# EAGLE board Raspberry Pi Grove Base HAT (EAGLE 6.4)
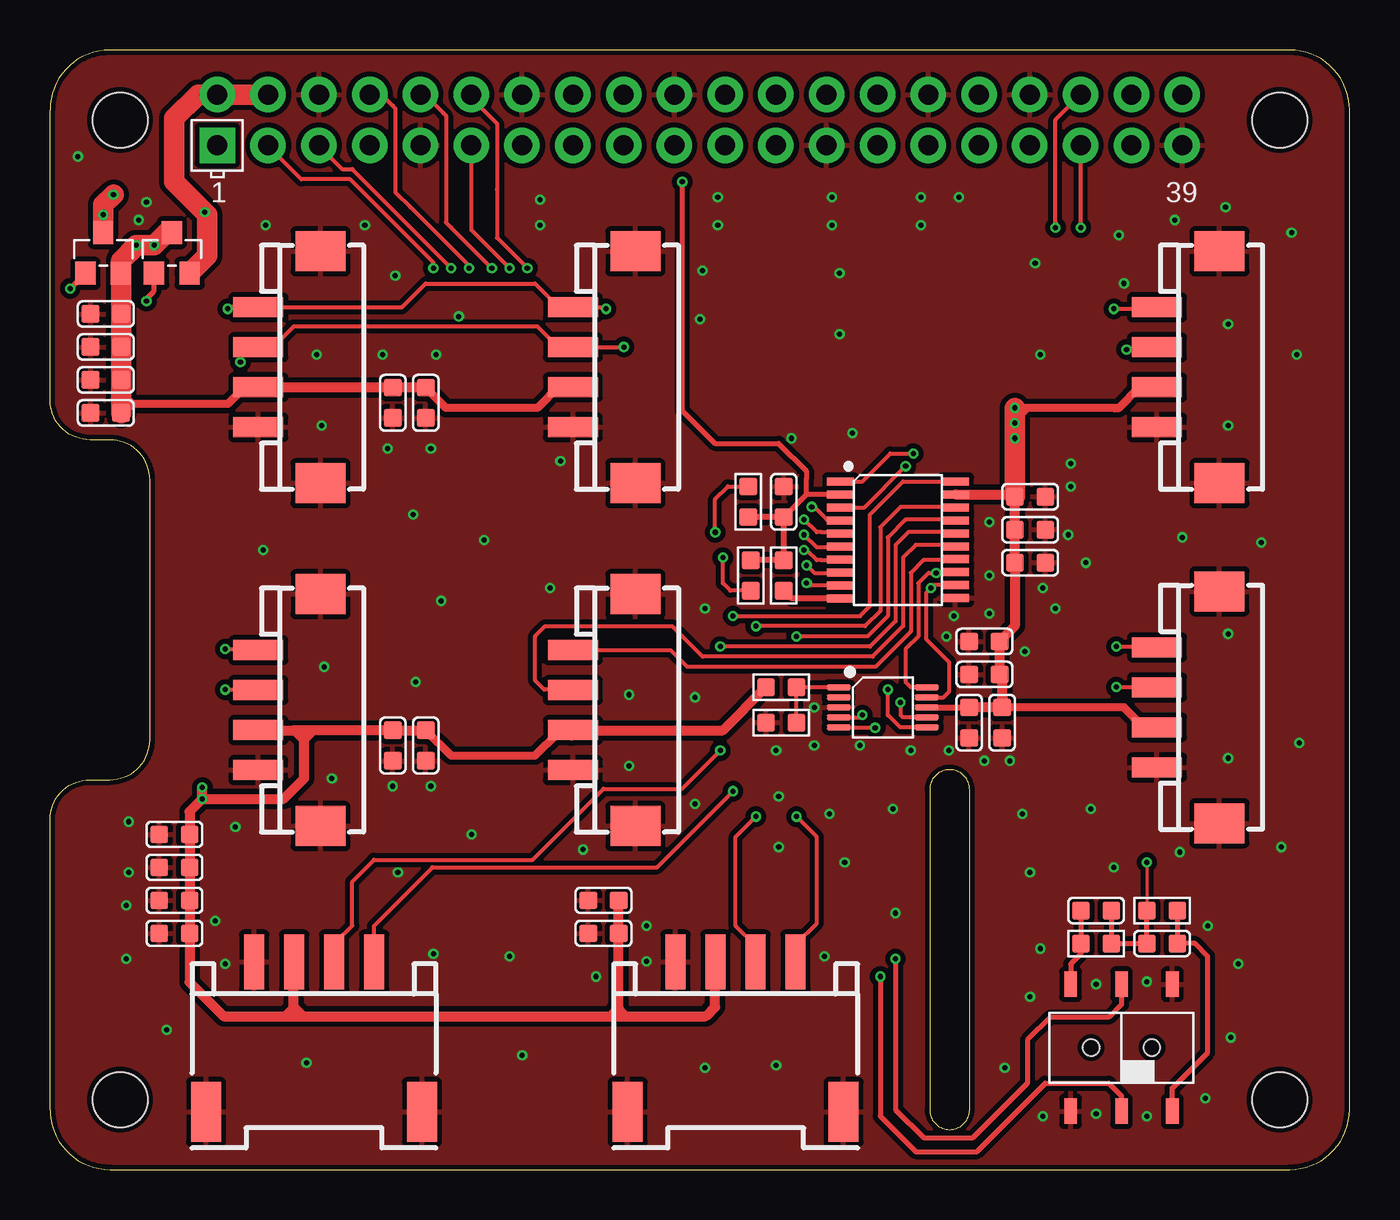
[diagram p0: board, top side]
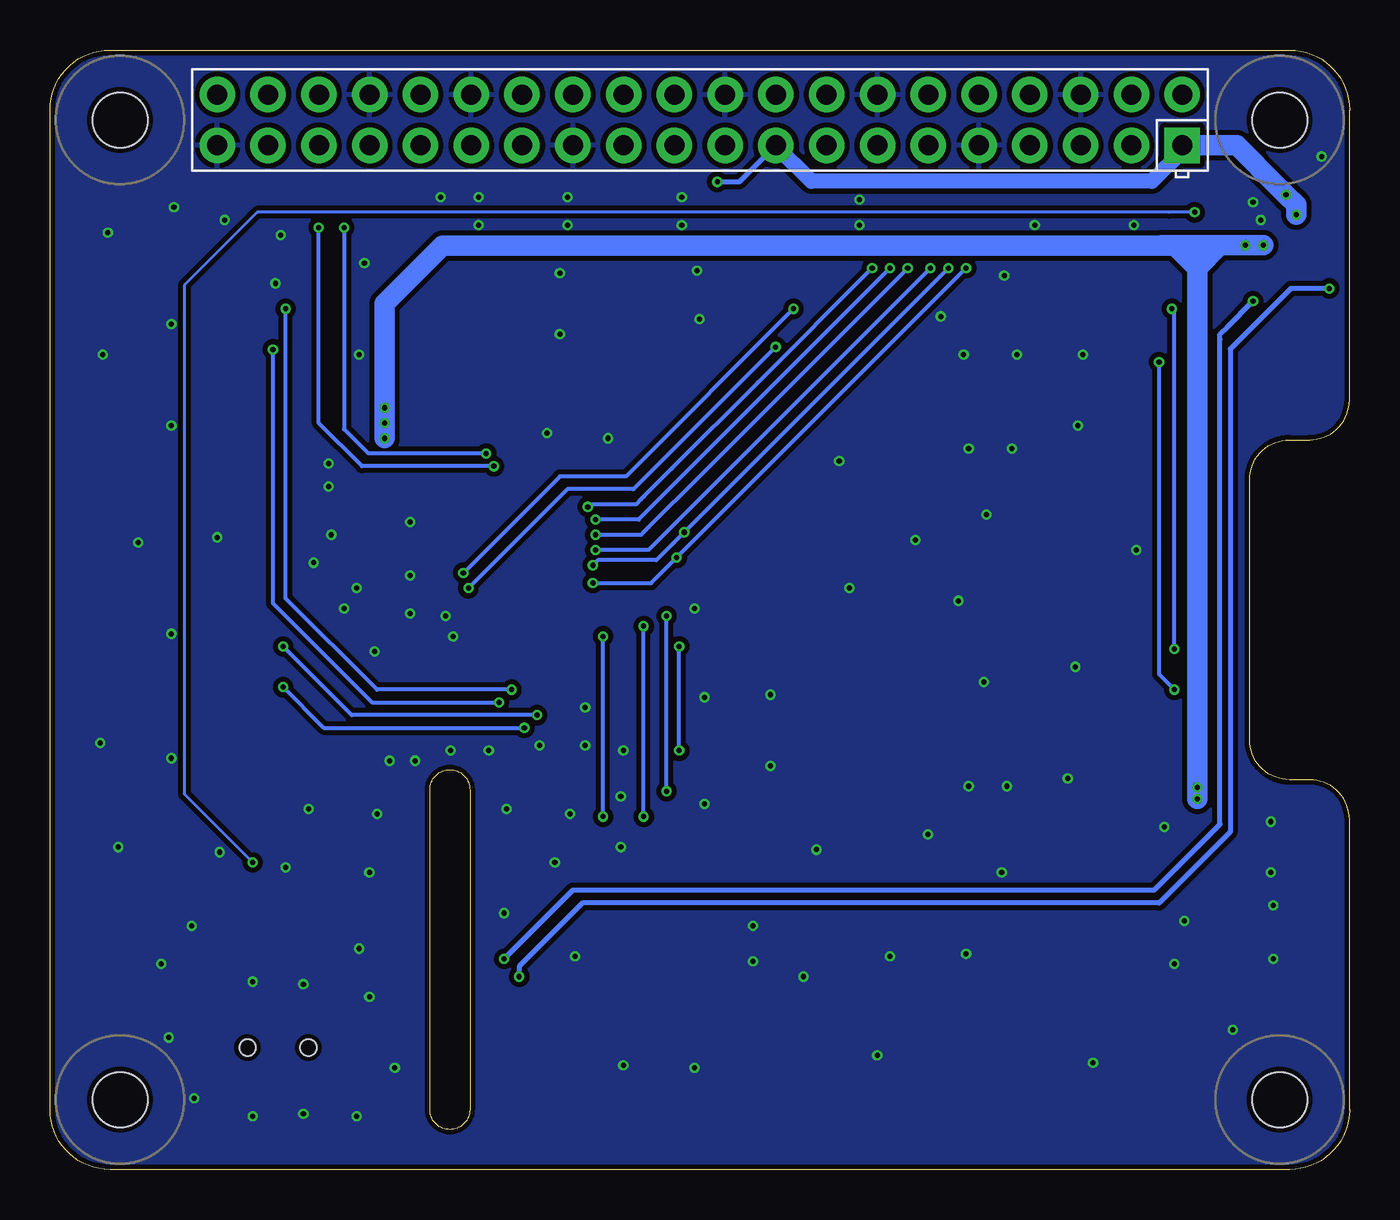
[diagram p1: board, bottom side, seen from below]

Size 65 x 56 mm. Coordinates in mm from the lower left corner, seen from the top.
Copper layers (1*16): Top 0.035mm / dielectric 1.5mm / Bottom 0.035mm
Design rules "SeeedStudio_2layer_DRU_no_angle_20140221 *": minimum track width 1mil, minimum drill 10mil, track to track 6mil, track to pad 6mil, pad to pad 6mil, via to via 6mil, smd to smd 0mil, copper to edge 10mil, drill to drill 10mil, minimum pad ring 4mil, minimum via ring 4mil, stop-mask expansion 2mil, vias tented up to drill 25mil, thermal gap 10mil
Net classes: 0 default: width 0.025 mm, clearance 0.152 mm

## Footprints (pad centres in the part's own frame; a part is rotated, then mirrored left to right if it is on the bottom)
C0603 = smd 0.889 x 0.889: 1 0,0.762; 2 0,-0.762
HW4-SMD-2.0 = smd 1 x 2.5: 1 -3,0; 2 -1,0; 3 1,0; 4 3,0 | smd 2 x 2.5: SS1 -5.8,3.123; SS2 5.8,3.123
HW4-SMD-2.0-90D = smd 1.01 x 2.74: 1 -3,-0.1; 2 -1,-0.1; 3 1,-0.1; 4 3,-0.1 | smd 1.5 x 3: SS1 -5.4,7.4; SS2 5.4,7.4
SOT-23 = smd 1.143 x 1.016: 1 1.016,-0.889; 2 1.016,0.889; 3 -1.016,0
R0603 = smd 0.889 x 0.889: 1 0,0.762; 2 0,-0.762
6P-SMD-2CH-2.54-3.5X7.2 = smd 1.27 x 0.635: CH1A -3.175,2.54; CH1B -3.175,-2.54; CH2A 3.175,2.54; CH2B 3.175,-2.54; COM1 -3.175,0; COM2 3.175,0 | hole 0.813: 0,1.524; 0,-1.524
SSOP10-0.5-3X3MM = smd 0.3 x 1.2: 1 -1,-2.2; 2 -0.5,-2.2; 3 0,-2.2; 4 0.5,-2.2; 5 1,-2.2; 6 1,2.2; 7 0.5,2.2; 8 0,2.2; 9 -0.5,2.2; 10 -1,2.2
RASPI_BOARD_B+HAT_DF_CF = drill 1 pad 1.778 square: 1 8.37,51.23 | drill 1 pad 1.778: 2 8.37,53.77; 3 10.91,51.23; 4 10.91,53.77; 5 13.45,51.23; 6 13.45,53.77; 7 15.99,51.23; 8 15.99,53.77; 9 18.53,51.23; 10 18.53,53.77; 11 21.07,51.23; 12 21.07,53.77; 13 23.61,51.23; 14 23.61,53.77; 15 26.15,51.23; 16 26.15,53.77; 17 28.69,51.23; 18 28.69,53.77; 19 31.23,51.23; 20 31.23,53.77; 21 33.77,51.23; 22 33.77,53.77; 23 36.31,51.23; 24 36.31,53.77; 25 38.85,51.23; 26 38.85,53.77; 27 41.39,51.23; 28 41.39,53.77; 29 43.93,51.23; 30 43.93,53.77; 31 46.47,51.23; 32 46.47,53.77; 33 49.01,51.23; 34 49.01,53.77; 35 51.55,51.23; 36 51.55,53.77; 37 54.09,51.23; 38 54.09,53.77; 39 56.63,51.23; 40 56.63,53.77 | hole 2.75: 3.5,3.5; 3.5,52.5; 61.5,3.5; 61.5,52.5
TSSOP20-0.65-6.5X4.4MM = smd 0.4 x 1.35: 1 -2.925,-2.875; 2 -2.275,-2.875; 3 -1.625,-2.875; 4 -0.975,-2.875; 5 -0.325,-2.875; 6 0.325,-2.875; 7 0.975,-2.875; 8 1.625,-2.875; 9 2.275,-2.875; 10 2.925,-2.875; 11 2.91,2.875; 12 2.26,2.875; 13 1.61,2.875; 14 0.96,2.875; 15 0.325,2.875; 16 -0.325,2.875; 17 -0.975,2.875; 18 -1.625,2.875; 19 -2.275,2.875; 20 -2.925,2.875

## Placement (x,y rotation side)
C1  DNP  [C0603]  47.63,22.35 180 top
C2  100nF  [C0603]  45.97,22.35 180 top
C3  100nF  [C0603]  2.79,37.85 90 top
C4  100nF  [C0603]  18.8,38.35 180 top
C5  1uF  [C0603]  2.79,39.5 90 top
C6  1uF  [C0603]  17.15,38.35 180 top
C7  100nF  [C0603]  46.74,24.77 90 top
C8  1uF  [C0603]  46.74,26.42 90 top
C9  100nF  [C0603]  49.02,32 270 top
C10  1uF  [C0603]  49.02,33.66 270 top
C11  100nF  [C0603]  6.22,15.11 90 top
C12  1uF  [C0603]  6.22,16.76 90 top
C13  100nF  [C0603]  18.8,21.21 180 top
C14  1uF  [C0603]  17.15,21.21 180 top
C15  100nF  [C0603]  6.22,11.81 90 top
C16  1uF  [C0603]  6.22,13.46 90 top
C17  100nF  [C0603]  27.69,11.81 90 top
C18  1uF  [C0603]  27.69,13.46 90 top
C19  100nF  [C0603]  36.7,33.4 0 top
C20  DNP  [C0603]  49.02,30.35 270 top
C21  100nF  [C0603]  2.79,41.15 90 top
C22  10uF  [C0603]  2.79,42.8 270 top
C23  100nF  [C0603]  52.32,12.95 90 top
C24  100nF  [C0603]  55.63,11.3 270 top
FR  SEEEDSTUDIO-OPEN-SCH-FRAME  [SEEEDSTUDIO-PCB-FRAME]  not placed on the board
FR1  SEEEDSTUDIO-OPEN-SCH-FRAME  [SEEEDSTUDIO-PCB-FRAME]  not placed on the board
J1  4P-2.0;320110030  [HW4-SMD-2.0]  10.41,40.13 270 top
J2  4P-2.0;320110030  [HW4-SMD-2.0]  26.16,40.13 270 top
J3  4P-2.0;320110030  [HW4-SMD-2.0]  55.37,23.11 270 top
J4  4P-2.0;320110030  [HW4-SMD-2.0]  55.37,40.13 270 top
J5  4P-2.0;320110030  [HW4-SMD-2.0]  10.41,22.99 270 top
J6  4P-2.0;320110030  [HW4-SMD-2.0]  26.16,22.99 270 top
J7  4P-2.0;320110030  [HW4-SMD-2.0-90D]  13.21,10.29 180 top
J8  4P-2.0;320110030  [HW4-SMD-2.0-90D]  34.29,10.29 180 top
Q3  CJ2305  [SOT-23]  2.67,45.85 270 top
Q4  CJ2305  [SOT-23]  6.1,45.85 270 top
R1  DNP  [R0603]  36.58,24.13 90 top
R2  0R  [R0603]  36.58,22.35 90 top
R3  4.7k  [R0603]  36.7,29.72 180 top
R4  DNP  [R0603]  34.93,33.4 0 top
R5  DNP  [R0603]  35.05,29.72 180 top
R13  100K  [R0603]  52.32,11.3 270 top
R14  100K  [R0603]  55.63,12.95 270 top
SW2  SWITCH-2CH-6P-2.54  [6P-SMD-2CH-2.54-3.5X7.2]  53.59,6.1 270 top
U1  ADS1015  [SSOP10-0.5-3X3MM]  41.66,23.11 270 top
U2  2x20 2.54  [RASPI_BOARD_B+HAT_DF_CF]  0,0 0 top
U3  TXS0108E  [TSSOP20-0.65-6.5X4.4MM]  42.42,31.5 270 top

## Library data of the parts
C1-C24 Q3 Q4 R1-R5 R13 R14 = Discrete-new
FR FR1 = moudle-new
J1-J8 = Connector-new
SW2 = Discrete
U1 = IC-new; MPN: ADS1015IDGST-ADC-兼容1.8V-3.3V
U2 U3 = IC-new

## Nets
3V3_RPI: C19.2 Q3.3 R3.2 R4.2 R5.2 U2.1 U2.17 U3.2
3V3_SIG: Q3.1 SW2.COM2
5V_RPI: C23.2 C24.2 Q4.2 R13.1 R14.2 U2.2 U2.4
5V_SIG: Q4.1 SW2.COM1
AIN0: J3.1 U1.4
AIN1: J3.2 U1.5
AIN2: J4.1 U1.6
AIN3: J4.2 U1.7
GND: C1.1 C2.1 C3.1 C4.1 C5.1 C6.1 C7.1 C8.1 C9.1 C10.1 C11.1 C12.1 C13.1 C14.1 C15.1 C16.1 C17.1 C18.1 C19.1 C20.1 C21.1 C22.2 J1.4 J1.SS1 J1.SS2 J2.4 J2.SS1 J2.SS2 J3.4 J3.SS1 J3.SS2 J4.4 J4.SS1 J4.SS2 J5.4 J5.SS1 J5.SS2 J6.4 J6.SS1 J6.SS2 J7.4 J7.SS1 J7.SS2 J8.4 J8.SS1 J8.SS2 R2.1 SW2.CH1A SW2.CH2B U1.3 U2.6 U2.9 U2.14 U2.20 U2.25 U2.30 U2.34 U2.39 U3.11
GPIO16_H: J7.1 U3.20
GPIO16_RPI: U2.36 U3.1
GPIO17_H: J7.2 U3.16
GPIO17_RPI: U2.11 U3.5
GPIO18_H: J8.1 U3.17
GPIO18_RPI: U2.12 U3.4
GPIO19_H: J8.2 U3.18
GPIO19_RPI: U2.35 U3.3
GROVE_POWER: C1.2 C2.2 C3.2 C4.2 C5.2 C6.2 C7.2 C8.2 C9.2 C10.2 C11.2 C12.2 C13.2 C14.2 C15.2 C16.2 C17.2 C18.2 C20.2 C21.2 C22.1 J1.3 J2.3 J3.3 J4.3 J5.3 J6.3 J7.3 J8.3 Q3.2 Q4.3 R1.1 U1.8 U3.19
N$2: R1.2 R2.2 U1.1
N$5: R3.1 U3.10
N$11: C23.1 R13.2 SW2.CH1B
N$15: C24.1 R14.1 SW2.CH2A
RX_H: J6.2 U3.15
RX_RPI: U2.10 U3.6
SCL_H: J1.1 J2.1 J5.1 U1.10 U3.13
SCL_RPI: R4.1 U2.5 U3.8
SDA_H: J1.2 J2.2 J5.2 U1.9 U3.12
SDA_RPI: R5.1 U2.3 U3.9
TX_H: J6.1 U3.14
TX_RPI: U2.8 U3.7

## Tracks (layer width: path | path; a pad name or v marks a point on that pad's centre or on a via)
3V3_RPI  (via drill 0.25 pad 0.51)
  Top 0.254: U3.2 37.84,33.77 | 37.84,33.77 C19.2 | 37.84,33.77 37.84,34.54 37.84,34.94 36.45,36.32 33.27,36.32 31.62,37.97 31.62,48.64 v31.62,49.4
  Top 0.305: R5.2 R3.2 C19.2 R4.2
  Top 1.016: v3.18,48.77 2.67,48.26 v2.67,47.75 Q3.3
  Bottom 0.254: U2.17 30.52,49.4 v31.62,49.4
  Bottom 0.762: U2.1 8.37,50.94 9.88,49.43 26.92,49.43 28.7,51.22 U2.17
  Bottom 1.016: U2.1 5.64,51.23 3.56,49.15 v3.18,48.77 2.67,48.26 v2.67,47.75
3V3_SIG  (via drill 0.25 pad 0.51)
  Top 0.254: Q3.1 v1.02,44.07 | v41.53,9.65 41.53,2.67 43.31,0.89 46.36,0.89 49.78,4.32 52.96,4.32 53.59,3.68 SW2.COM2
  Bottom 0.254: v1.02,44.07 2.94,44.07 5.97,41.04 5.97,16.87 5.99,16.87 9.53,13.34 38.35,13.34 41.53,10.16 v41.53,9.65
5V_RPI  (via drill 0.25 pad 0.51)
  Top 0.152: v54.86,15.37 R14.2
  Top 0.254: C23.2 R13.1 C24.2 R14.2
  Top 1.016: U2.4 U2.2 7.42,53.77 6.22,52.58 6.22,49.4 v7.75,47.88 7.87,47.75 7.87,45.72 Q4.2
  Bottom 0.152: v7.75,47.88 9.02,47.88 54.63,47.88 58.28,44.23 58.28,18.78 v54.86,15.37
5V_SIG  (via drill 0.25 pad 0.51)
  Top 0.254: SW2.COM1 53.59,8.26 52.96,7.62 50.04,7.62 48.9,6.48 48.9,4.32 46.17,1.59 43.7,1.59 42.29,3 v42.29,10.54 | v4.83,43.43 4.83,43.56 5.21,43.94 Q4.1
  Bottom 0.254: v42.29,10.54 38.86,13.97 9.78,13.97 6.48,17.27 6.48,41.53 6.48,41.78 6.1,42.16 v4.83,43.43
AIN0  (via drill 0.25 pad 0.51)
  Top 0.203: U1.4 40.52,22.61 v40.64,22.73 | v53.34,26.16 55.32,26.16 J3.1
  Bottom 0.203: v40.64,22.73 49.91,22.73 v53.34,26.16
AIN1  (via drill 0.25 pad 0.51)
  Top 0.203: U1.5 41.26,22.11 v41.28,22.1 | 55.23,24.26 J3.2 55.36,24.13 v53.34,24.13
  Bottom 0.203: v53.34,24.13 51.31,22.1 v41.28,22.1
AIN2  (via drill 0.25 pad 0.51)
  Top 0.203: U1.6 42.53,22.11 41.91,22.73 v41.91,24 | v53.21,43.05 55.29,43.05 J4.1
  Bottom 0.203: v53.21,43.05 53.21,28.57 48.64,24 v41.91,24
AIN3  (via drill 0.25 pad 0.51)
  Top 0.203: U1.7 42.66,22.61 42.55,22.73 v42.55,23.37 | 55.36,41.15 J4.2 55.26,41.02 v53.85,41.02
  Bottom 0.203: v53.85,41.02 53.85,28.32 48.9,23.37 v42.55,23.37
GND  (via drill 0.25 pad 0.51)
  other vias: 12.83,5.33 23.62,5.72 32.77,5.08 36.32,5.21 19.18,10.8 22.99,10.67 44.96,20.95 46.74,20.45 48.01,20.45 44.83,26.67 45.21,27.69 46.99,27.81 46.99,29.72 46.99,32.39 48.77,25.91 50.29,28.07 49.66,29.08 51.82,30.35 50.93,31.75 51.05,34.16 51.05,35.31 49.53,40.77 53.47,46.74 53.72,44.32 49.28,45.34 58.8,48.13 56.26,47.5 62.1,46.86 62.36,40.77 58.93,42.29 58.93,37.21 56.64,31.62 60.58,31.37 58.93,26.8 58.93,20.57 62.48,21.34 53.21,15.11 49.02,14.86 49.53,11.05 56.52,15.88 61.6,16.13 57.91,12.19 54.86,9.4 52.32,9.27 59.44,10.29 59.06,6.6 57.79,3.56 54.86,2.67 52.32,2.79 49.66,2.67 47.75,5.08 49.02,8.64 48.64,17.78 52.07,18.03 38.23,23.11 38.23,21.21 40.51,21.21 43.05,20.95 36.32,20.95 36.45,18.67 36.45,16.13 38.99,17.78 42.16,18.03 39.75,15.37 42.29,12.83 38.74,10.67 29.85,12.19 29.85,10.41 27.31,9.65 8.26,12.45 8.76,10.29 9.27,17.15 17.15,19.18 19.05,19.18 14.1,19.56 21.08,16.76 32.26,18.29 26.67,16 28.96,20.19 32.26,23.62 28.96,23.75 32.77,28.07 25.02,29.08 25.53,35.43 16.89,36.07 37.08,36.58 13.59,37.21 10.67,30.99 18.16,32.77 13.72,25.15 18.29,24.38 21.72,31.5 17.27,44.7 32.51,42.55 39.5,41.78 3.94,17.4 3.94,14.86 3.81,13.21 3.81,10.54 5.84,6.98 19.05,36.07 19.56,28.45 13.34,40.77 19.3,40.77 40.13,36.83 39.5,44.83 32.64,44.96 45.47,48.64 39.12,47.24 43.56,47.24 33.4,47.24 24.51,47.24 10.8,47.24 15.75,47.24 4.83,48.39 1.4,50.67 43.56,48.64 39.12,48.64 33.4,48.64 24.51,48.51 4.45,47.5 17.4,14.86 20.45,42.67 16.64,40.77
  pour Top (isolate 0.254, rank 6): -0.63,56.39 65.41,56.39 65.41,-0.25 -0.63,-0.25
  pour Bottom (isolate 0.254, rank 6): -1.02,56.64 65.66,56.64 65.66,-0.51 -1.02,-0.51
GPIO16_H  (via drill 0.25 pad 0.51)
  Top 0.203: J7.1 16.21,12.19 19.13,15.11 30.35,15.11 v34.16,18.92 | U3.20 42.67,34.42 41.02,32.77 41.02,28.19 40.51,27.69 v34.16,27.69
  Bottom 0.203: v34.16,18.92 v34.16,27.69
GPIO16_RPI  (via drill 0.25 pad 0.51)
  Top 0.203: U2.36 50.29,52.51 50.29,47.37 v50.29,47.12 | U3.1 40.64,34.42 42.04,35.81 v43.18,35.81
  Bottom 0.203: v43.18,35.81 49.07,35.81 50.06,36.81 50.29,37.04 v50.29,47.12
GPIO17_H  (via drill 0.25 pad 0.51)
  Top 0.203: J7.2 14.32,10.39 14.32,11.4 15.11,12.19 15.11,14.4 16.21,15.49 24.13,15.49 27.69,19.05 31.62,19.05 v33.53,20.95 | U3.16 45.24,31.88 42.93,31.88 42.29,31.24 42.29,27.43 41.02,26.16 v33.53,26.16
  Bottom 0.203: v33.53,20.95 v33.53,26.16
GPIO17_RPI  (via drill 0.25 pad 0.51)
  Top 0.203: U2.11 21.07,49.16 21.07,47 v22.99,45.09 | U3.5 39.49,31.88 38.61,31.88 38.35,31.88 v37.72,32.51
  Bottom 0.203: v22.99,45.09 29.08,38.99 33.78,34.29 35.05,33.02 35.31,32.77 35.43,32.64 35.56,32.51 v37.72,32.51
GPIO18_H  (via drill 0.25 pad 0.51)
  Top 0.203: U3.17 45.25,32.51 42.8,32.51 41.91,31.62 41.91,27.69 40.89,26.67 v37.34,26.67 | J8.1 37.34,10.44 37.34,11.3 38.35,12.32 38.35,16.64 v37.34,17.65
  Bottom 0.203: v37.34,17.65 v37.34,26.67
GPIO18_RPI  (via drill 0.25 pad 0.51)
  Top 0.203: U2.12 21.07,53.61 22.35,52.32 22.35,49.02 22.35,46.61 v23.88,45.09 | v38.1,33.15 38.23,33.15 38.86,32.51 39.5,32.51 U3.4
  Bottom 0.203: v23.88,45.09 29.59,39.37 33.91,35.05 35.31,33.66 35.43,33.53 35.69,33.27 37.97,33.27 v38.1,33.15
GPIO19_H  (via drill 0.25 pad 0.51)
  Top 0.203: U3.18 45.27,33.15 42.55,33.15 41.53,32.13 41.53,27.94 40.77,27.18 v35.31,27.18 | J8.2 35.31,10.4 35.31,11.18 34.29,12.19 34.29,16.64 v35.31,17.65
  Bottom 0.203: v35.31,17.65 v35.31,27.18
GPIO19_RPI  (via drill 0.25 pad 0.51)
  Top 0.203: U3.3 40.74,33.12 v42.8,35.18 | v51.56,47.12 51.55,47.13 U2.35
  Bottom 0.203: v42.8,35.18 49.4,35.18 51.56,37.34 v51.56,47.12
GROVE_POWER  (via drill 0.25 pad 0.51)
  Top 0.203: 10.3,39.37 10.3,39.26 10.29,39.24 10.41,39.24 10.54,39.12 | 26.18,21.97 J6.3 26.16,21.72 | 3.56,38.73 3.81,38.73 4.19,38.35 4.19,38.23 3.94,37.97 | 48.26,37.72 48.64,37.72 49.02,38.1
  Top 0.254: U1.8 43.94,23.11 | 26.04,21.72 26.16,21.72 26.8,21.72
  Top 0.305: 43.94,23.11 C2.2
  Top 0.406: 12.19,21.97 12.57,21.59 12.83,21.59 13.08,21.84 | 9.78,38.99 9.59,38.99 8.89,38.29 3.62,38.29 | C13.2 20.07,20.7 24.26,20.7 25.4,21.84 26.02,21.84 J6.3 | 47.75,23.49 47.63,23.62 | J2.3 25.42,39.13 24.38,38.1 19.81,38.1 C4.2 | J3.3 54.72,22.11 53.72,23.11 C1.2 | v48.26,38.1 49.02,38.1 53.2,38.1 53.34,38.1 53.47,38.1 54.5,39.13 J4.3
  Top 0.508: J5.3 10.43,21.97 12.19,21.97 12.7,21.97 | 26.04,21.72 26.15,21.72 | C13.2 C14.2 12.7,21.97 | 11.76,7.66 12.19,8.1 12.19,8.13 | 12.19,8.13 12.19,10.37 J7.3 | 12.66,7.66 28.03,7.66 | 28.03,7.66 28.45,8.09 C17.2 C18.2 | 11.76,7.66 12.66,7.66 | 12.66,7.66 12.19,8.13 | 28.03,7.66 28.79,7.66 | 28.79,7.66 32.81,7.66 33.27,8.13 33.27,10.37 J8.3 | 28.79,7.66 28.45,8 | v7.62,18.54 6.99,17.91 C12.2 C11.2 C16.2 C15.2 6.99,9.37 8.69,7.66 11.76,7.66 | v7.62,18.54 v7.62,19.11 | C10.2 48.26,33.78 | U3.19 48.14,33.77 C10.2 | C10.2 C9.2 C20.2 48.26,27.18 C8.2 C7.2 47.63,24.64 47.63,23.62 C1.2 C2.2 | 11.76,7.66 | C4.2 C6.2 10.54,39.12 9.91,39.12 9.78,38.99 10.27,38.99 J1.3 | 26.18,21.97 33.66,21.97 R1.1 | v7.62,18.54 11.68,18.54 12.7,19.56 12.7,21.97
  Top 1.016: v48.26,38.1 48.26,37.72 v48.26,36.58 C10.2 | Q4.3 5.84,46.86 v5.21,46.23 v4.32,46.23 3.94,45.85 3.56,45.47 Q3.2 C22.1 C21.2 C5.2 3.56,38.73 C3.2 3.56,38.23 3.62,38.29
  Bottom 1.016: v48.26,36.58 v48.26,37.34 v48.26,38.1 48.26,43.31 45.35,46.22 8.75,46.22 8.64,46.1 7.81,45.28 7.62,45.09 | v7.62,18.54 v7.62,19.11 7.62,44.07 7.62,44.96 | 7.62,44.96 7.62,45.09 | v4.32,46.23 v5.21,46.23 6.48,46.23 | 6.48,46.23 6.86,46.23 9.4,46.23 | 7.62,44.96 7.62,45.09 | 7.62,45.09 6.48,46.23
N$2
  Top 0.203: R2.2 R1.2 39.44,24.13 U1.1
N$5
  Top 0.305: U3.10 37.09,28.57 R3.1
N$11
  Top 0.254: C23.1 R13.2 51.56,10.8 51.05,10.29 SW2.CH1B
N$15
  Top 0.254: R14.1 C24.1 57.28,11.3 57.91,10.67 57.91,5.84 56.13,4.06 SW2.CH2A
RX_H
  Top 0.203: U3.15 45.22,31.24 43.31,31.24 42.67,30.61 42.67,27.18 41.15,25.65 32.64,25.65 31.12,27.18 24.77,27.18 24.27,26.69 24.27,24.45 24.72,24 26.16,24 | 26.15,24 J6.2 26.18,24 26.16,24 | 25.04,23.73 25.89,23.73 26.16,24
RX_RPI  (via drill 0.25 pad 0.51)
  Top 0.203: U2.10 18.75,53.77 19.69,52.83 19.81,52.7 19.81,47.37 20.07,47.12 v22.1,45.09 | U3.6 39.49,31.11 38.35,31.11 v37.72,31.75
  Bottom 0.203: v22.1,45.09 32.51,34.67 35.05,32.13 35.18,32 35.31,31.88 35.43,31.75 v37.72,31.75
SCL_H  (via drill 0.25 pad 0.51)
  Top 0.203: 26.04,43.26 J2.1 | v44.32,29.84 43.94,29.84 43.43,29.34 43.43,26.67 42.8,26.04 42.8,24.38 43.07,24.11 U1.10 | v44.32,29.84 45.25,29.84 U3.13 45.38,29.97 45.85,29.97 45.72,29.84 v44.32,29.84 | v8.76,26.04 10.37,26.04 J5.1 | J2.1 27.73,43.13 v27.81,43.05 | v8.89,43.05 8.97,43.13 J1.1 17.61,43.13 18.8,44.32 24.26,44.32 25.27,43.31 25.99,43.31 J2.1
  Bottom 0.203: v27.81,43.05 36.2,34.67 39.5,34.67 v44.32,29.84 | v8.76,26.04 8.76,42.93 v8.89,43.05
SCL_RPI  (via drill 0.25 pad 0.51)
  Top 0.203: v20.07,45.09 18.48,46.67 16.64,48.51 15.11,50.04 14.61,50.04 13.45,51.19 U2.5 | U3.8 39.52,29.84 38.23,29.84 v37.85,30.23 | v33.27,31.88 33.27,33.53 33.91,34.16 R4.1
  Bottom 0.203: v20.07,45.09 v33.27,31.88 34.67,30.48 37.59,30.48 v37.85,30.23
SDA_H  (via drill 0.25 pad 0.51)
  Top 0.203: J5.2 8.78,23.99 v8.76,24 | v9.53,40.39 9.53,41.02 9.65,41.15 10.4,41.15 J1.2 10.65,40.89 10.92,40.89 12.19,42.16 24.38,42.16 25.42,41.13 J2.2 28.69,41.13 v28.7,41.15 | U3.12 44.22,29.24 v44.07,29.08 43.82,28.83 43.82,26.54 44.96,25.4 44.96,23.88 44.7,23.61 U1.9
  Bottom 0.203: v8.76,24 9.53,24.77 v9.53,40.39 | v28.7,41.15 35.81,34.04 39.12,34.04 v44.07,29.08
SDA_RPI  (via drill 0.25 pad 0.51)
  Top 0.203: v19.18,45.09 19.18,45.21 19.18,45.37 15.02,49.53 12.57,49.53 10.91,51.19 U2.3 | U3.9 39.53,29.21 37.97,29.21 v37.85,29.34 | R5.1 34.04,28.96 33.66,29.34 v33.66,30.61
  Bottom 0.203: v19.18,45.09 v33.66,30.61 34.93,29.34 v37.85,29.34
TX_H
  Top 0.203: U3.14 45.24,30.48 43.69,30.48 43.05,29.84 43.05,26.92 41.28,25.15 31.88,25.15 31.56,25.46 31.12,25.91 31.04,25.99 J6.1 26.46,26.29
TX_RPI  (via drill 0.25 pad 0.51)
  Top 0.203: U2.8 16.59,53.77 17.15,53.21 17.27,53.09 17.27,48.9 18.03,48.13 20.96,45.21 v20.96,45.09 | U3.7 39.5,30.48 38.61,30.48 38.35,30.48 37.85,30.99 v37.72,30.99
  Bottom 0.203: v37.72,30.99 37.59,30.99 37.47,30.99 35.05,30.99 22.35,43.69 22.23,43.81 v20.96,45.09

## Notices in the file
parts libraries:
moudle-new: This work is licensed under the Creative Commons Attribution 4.0 International License.
To view a copy of this license,visit:
http://creativecommons.org/licenses/by-sa/4.0
